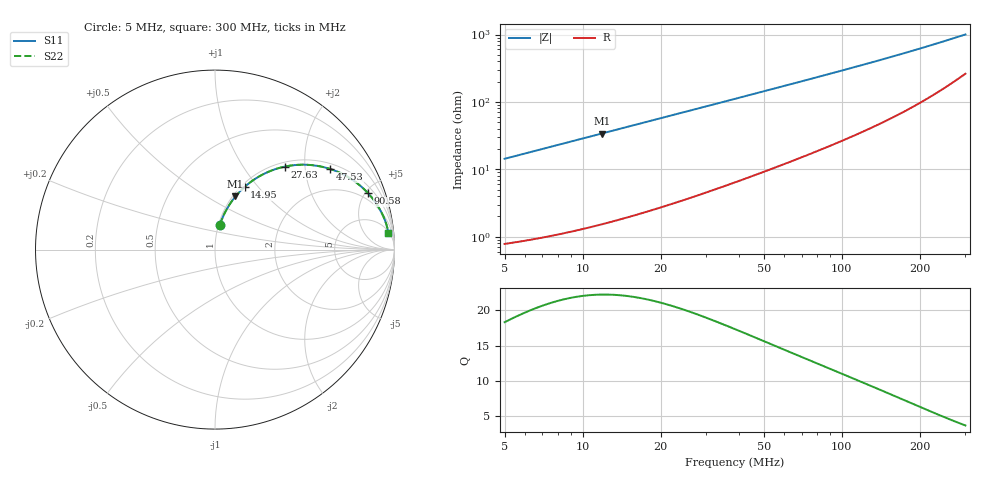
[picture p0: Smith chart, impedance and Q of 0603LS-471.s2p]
# MHz S MA R 50
!Freq  MagS11  AngS11  MagS21  AngS21  MagS12  AngS12  MagS22  AngS22
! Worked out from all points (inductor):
!   801 points, 5 MHz to 300 MHz, reference 50 ohm
!   read as one part in series: L = 455 nH near 5.103 MHz
!   highest Q = 22.2 at 11.87 MHz (marker M1), where L = 455 nH
!   S11 on the Smith chart (normalised r, x): 5 MHz: 1.02, +0.29; 14.95 MHz: 1.04, +0.85; 27.63 MHz: 1.08, +1.58; 47.53 MHz: 1.17, +2.72; 90.58 MHz: 1.45, +5.24; 300 MHz: 6, +19
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5  0.1406 78.8  0.9824 -8.1  0.9824 -8.1  0.1406 78.8
6.458095  0.1801 76.8  0.9748 -10.4  0.9748 -10.4  0.1801 76.8
8.006771  0.221 74.6  0.965 -12.8  0.965 -12.8  0.221 74.6
9.825733  0.2674 71.9  0.9515 -15.5  0.9515 -15.5  0.2674 71.9
11.8742  0.3172 68.9  0.9342 -18.5  0.9342 -18.5  0.3172 68.9
14.94946  0.3868 64.7  0.9048 -22.7  0.9048 -22.7  0.3868 64.7
17.60968  0.4417 61.2  0.877 -26.2  0.877 -26.2  0.4417 61.2
20.63739  0.498 57.4  0.8437 -29.8  0.8437 -29.8  0.498 57.4
27.62792  0.6053 49.9  0.7655 -37.2  0.7655 -37.2  0.6053 49.9
32.21283  0.6604 45.6  0.7161 -41.3  0.7161 -41.3  0.6604 45.6
37.36688  0.7109 41.5  0.6641 -45.2  0.6641 -45.2  0.7109 41.5
47.5284  0.7834 35.0  0.5745 -51.4  0.5745 -51.4  0.7834 35.0
54.29291  0.8177 31.5  0.5242 -54.7  0.5242 -54.7  0.8177 31.5
62.02018  0.8474 28.3  0.4747 -57.7  0.4747 -57.7  0.8474 28.3
70.48558  0.8719 25.3  0.4288 -60.4  0.4288 -60.4  0.8719 25.3
90.57577  0.9093 20.1  0.3457 -65.0  0.3457 -65.0  0.9093 20.1
103.467  0.9242 17.7  0.3061 -67.0  0.3061 -67.0  0.9242 17.7
125.6794  0.941 14.6  0.2539 -69.4  0.2539 -69.4  0.941 14.6
152.6604  0.953 12.0  0.2086 -71.1  0.2086 -71.1  0.953 12.0
202.2899  0.964 8.8  0.1541 -72.2  0.1541 -72.2  0.964 8.8
252.0866  0.9686 6.7  0.1196 -71.5  0.1196 -71.5  0.9686 6.7
300  0.9703 5.4  0.09689 -69.5  0.09689 -69.5  0.9703 5.4
